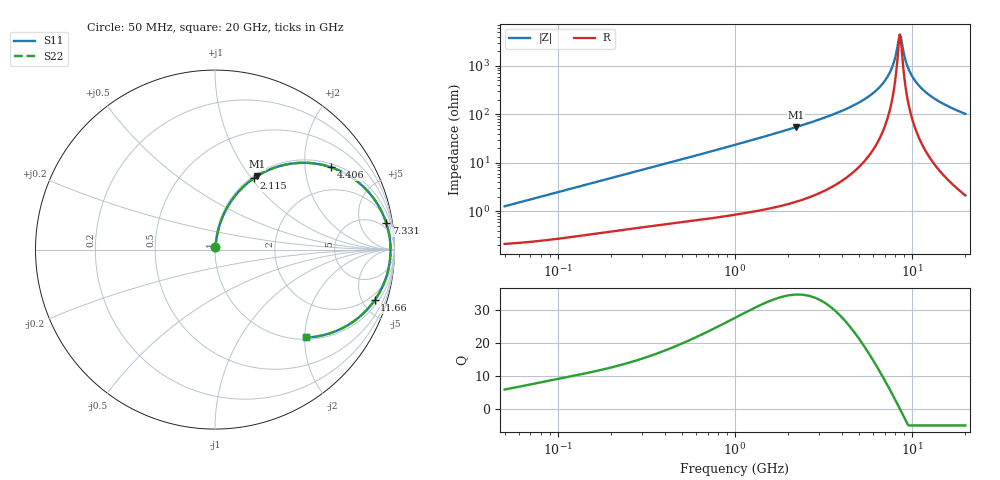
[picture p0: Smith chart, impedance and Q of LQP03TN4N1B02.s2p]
!Murata Part Number: LQP03TN4N1B02
!These Parameters are Measured in Series Mode Connection
!  o--[Z]--o
!Port1  Port2
!  o-------o
!Freq. Start=50[MHz] Stop=20[GHz], 401[Steps]
# Hz S RI R 50
!Freq.(Hz) S11(Real) S11(Imag) S21(Real) S21(Imag) S12(Real) S12(Imag) S22(Real) S22(Imag)
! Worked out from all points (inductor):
!   401 points, 50 MHz to 20 GHz, reference 50 ohm
!   read as one part in series: L = 3.96 nH near 51.52 MHz
!   highest Q = 34.7 at 2.212 GHz (marker M1), where L = 3.91 nH
!   self-resonance near 8.516 GHz
!   S11 on the Smith chart (normalised r, x): 50 MHz: 1.00, +0.02; 2.115 GHz: 1.03, +1.03; 4.406 GHz: 1.11, +2.74; 7.331 GHz: 3, +12; 11.66 GHz: 1.40, -6.14; 20 GHz: 1.04, -2.04
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5e7  0.00227 0.0124  0.9977 -0.0124  0.9977 -0.0124  0.00227 0.0124
1.364002e8  0.00423 0.033  0.9958 -0.033  0.9958 -0.033  0.00423 0.033
3.721004e8  0.0127 0.0863  0.9873 -0.0863  0.9873 -0.0863  0.0127 0.0863
1e9  0.0591 0.2184  0.9409 -0.2184  0.9409 -0.2184  0.0591 0.2184
2.114743e9  0.2171 0.3981  0.7829 -0.3981  0.7829 -0.3981  0.2171 0.3981
2.211938e9  0.2343 0.4094  0.7657 -0.4094  0.7657 -0.4094  0.2343 0.4094
2.728004e9  0.3305 0.4559  0.6695 -0.4559  0.6695 -0.4559  0.3305 0.4559
4.405649e9  0.6472 0.4585  0.3528 -0.4585  0.3528 -0.4585  0.6472 0.4585
6.034176e9  0.8669 0.3074  0.1331 -0.3074  0.1331 -0.3074  0.8669 0.3074
6.701223e9  0.9213 0.226  0.0787 -0.226  0.0787 -0.226  0.9213 0.226
7.331367e9  0.9547 0.1467  0.0453 -0.1467  0.0453 -0.1467  0.9547 0.1467
7.442007e9  0.959 0.1329  0.041 -0.1329  0.041 -0.1329  0.959 0.1329
7.901521e9  0.9718 0.076  0.0282 -0.076  0.0282 -0.076  0.9718 0.076
8.389408e9  0.9777 0.0177  0.0223 -0.0177  0.0223 -0.0177  0.9777 0.0177
8.516016e9  0.9781 0.00302  0.0219 -0.00302  0.0219 -0.00302  0.9781 0.00302
8.774992e9  0.9775 -0.0263  0.0225 0.0263  0.0225 0.0263  0.9775 -0.0263
9.178299e9  0.9734 -0.0702  0.0266 0.0702  0.0266 0.0702  0.9734 -0.0702
9.745021e9  0.9617 -0.1274  0.0383 0.1274  0.0383 0.1274  0.9617 -0.1274
1.050288e10  0.938 -0.1958  0.062 0.1958  0.062 0.1958  0.938 -0.1958
1.166392e10  0.8894 -0.2825  0.1106 0.2825  0.1106 0.2825  0.8894 -0.2825
1.460232e10  0.7429 -0.4194  0.2571 0.4194  0.2571 0.4194  0.7429 -0.4194
2e10  0.5092 -0.4896  0.4908 0.4896  0.4908 0.4896  0.5092 -0.4896
